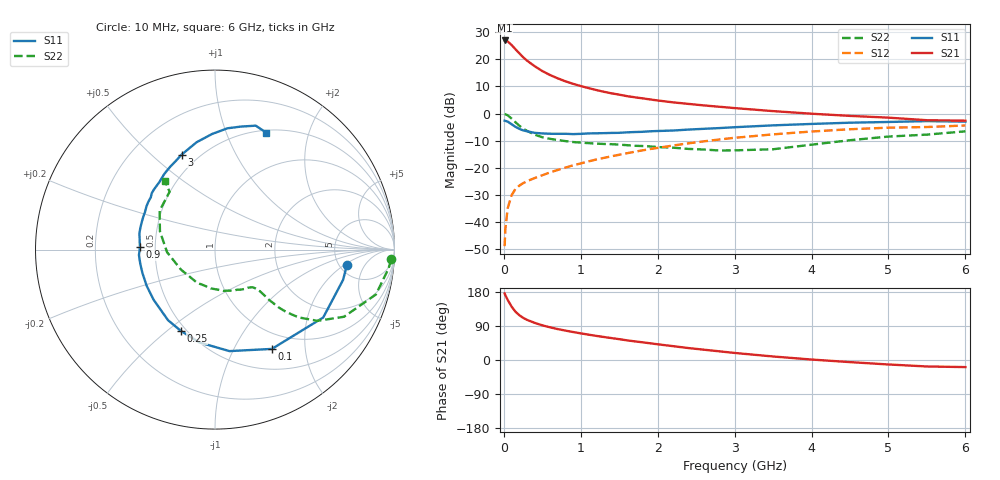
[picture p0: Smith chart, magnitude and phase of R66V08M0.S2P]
! SIEMENS Small Signal Semiconductors
! BFR193
! Si NPN RF Bipolar Junction Transistor in SOT23
! VCE = 6 V  IC = 8 mA
! Common Emitter S-Parameters:  May  1996
# GHz  S  MA  R  50
!  f  S11  S21  S12  S22
! GHz  MAG  ANG  MAG  ANG  MAG  ANG  MAG  ANG
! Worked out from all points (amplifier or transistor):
!   36 points, 10 MHz to 6 GHz, reference 50 ohm
!   highest |S21| = 27.0 dB at 10 MHz (marker M1)
!   |S21| within 3 dB of that: start of sweep to 143.5 MHz
!   unconditionally stable (mu >= 1): 809.5 MHz to 2.011 GHz
!   at 250 MHz: K = 0.57, MSG = 23.2 dB, |S12| = -25.7 dB
!   at 1.4 GHz: K = 1.05, MAG = 10.3 dB, |S12| = -15.7 dB
!   at 6 GHz: K = 0.95, MSG = 0.9 dB, |S12| = -4.4 dB
!   lowest NFmin = 1.25 dB at 450 MHz
!   S11 on the Smith chart (normalised r, x): 10 MHz: 5.79, -2.24; 100 MHz: 0.77, -1.43; 250 MHz: 0.47, -0.56; 900 MHz: 0.41, +0.01; 3 GHz: 0.41, +0.63; 6 GHz: 0.53, +1.39
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0.01  0.7397 -6.8  22.29 175.6  0.0036 90.2  0.9845 -3.2
0.02  0.7333 -13.3  22.01 170.9  0.0075 83.8  0.9717 -6.4
0.05  0.7118 -32.1  21.36 158.6  0.0179 75.2  0.9305 -15.6
0.1  0.6376 -60.2  18.43 141.2  0.0311 64.6  0.8103 -27.5
0.15  0.5713 -81.9  15.41 127.7  0.0407 57.9  0.6954 -34.8
0.2  0.5242 -99.8  12.99 118.4  0.0469 55.1  0.6003 -39.0
0.25  0.491 -112.9  10.97 111.4  0.0521 53.7  0.529 -41.2
0.3  0.4726 -123.6  9.501 106.0  0.0566 53.4  0.481 -42.2
0.4  0.4417 -140.8  7.486 98.0  0.0648 54.3  0.4103 -42.9
0.5  0.4309 -152.1  6.082 91.5  0.073 56.0  0.3665 -42.8
0.6  0.4249 -161.9  5.144 86.3  0.0824 57.4  0.3427 -42.8
0.7  0.4238 -169.1  4.466 81.6  0.0913 58.7  0.3258 -43.3
0.9  0.4186 178.2  3.539 73.8  0.1111 60.5  0.299 -44.7
1.1  0.4311 167.8  2.953 66.9  0.1315 61.2  0.2855 -47.8
1.3  0.4361 159.2  2.525 60.7  0.1526 61.0  0.2756 -51.3
1.6  0.4512 147.9  2.098 51.9  0.1858 60.1  0.2618 -58.6
2.2  0.4874 129.5  1.611 36.5  0.2581 55.5  0.2354 -77.9
3  0.5609 109.4  1.263 18.6  0.3579 45.6  0.2101 -118.1
3.5  0.6069 99.7  1.111 9.3  0.4144 38.2  0.2201 -149.6
4.5  0.6796 84.1  0.907 -5.6  0.5148 22.8  0.3231 161.7
5.5  0.7268 71.8  0.755 -17.1  0.5654 6.9  0.4097 128.1
6  0.7114 66.3  0.74 -18.7  0.6039 2.2  0.471 126.3
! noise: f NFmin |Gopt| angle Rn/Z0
0.45  1.25  0.23  133  0.12
0.9  1.3  0.35  156  0.11
1.8  2  0.55  -155  0.13
